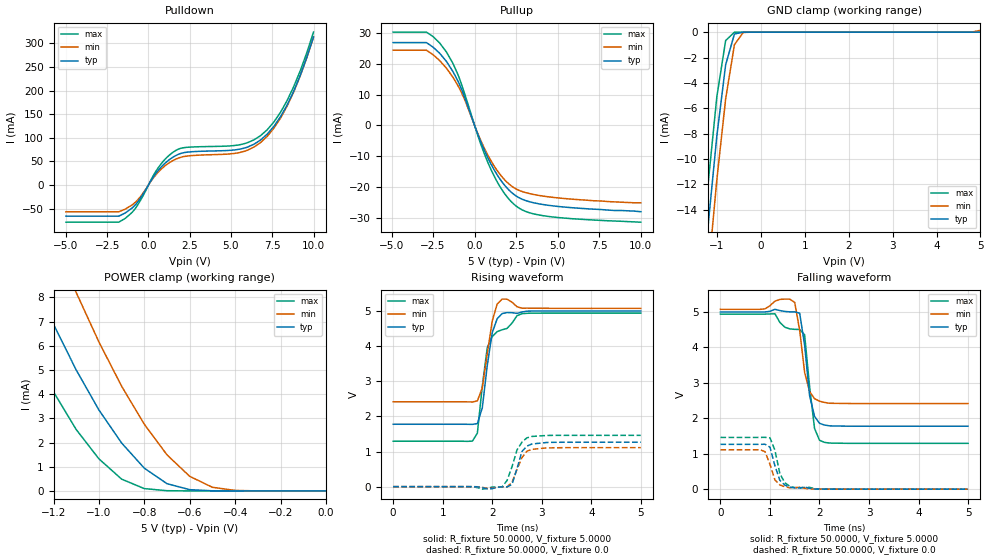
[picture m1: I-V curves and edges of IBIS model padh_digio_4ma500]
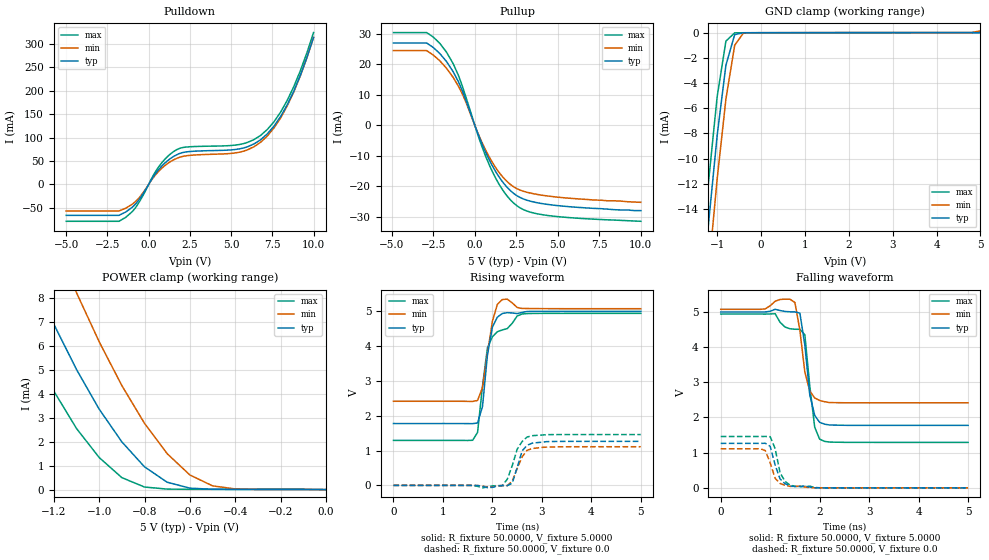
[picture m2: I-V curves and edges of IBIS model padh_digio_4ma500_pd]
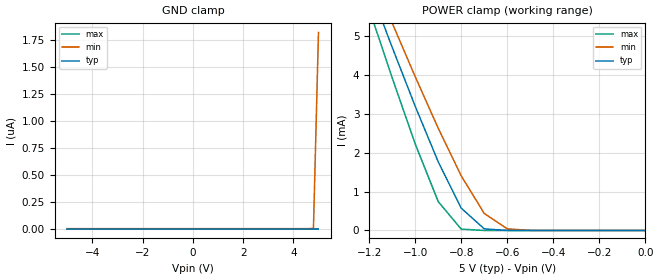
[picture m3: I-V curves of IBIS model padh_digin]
| IBIS file cs4272.ibs created by s2ibis3 verion 1.0
| North Carolina State University, ERL, 2005
[IBIS ver]   3.2
[Comment char]  |_char
[File name]   cs4272.ibs
[File Rev]   1.0B
[Date]   January 26, 2003
[Source]   HSpice Netlist
[Notes]   Rev. 1.0  1/26/2006  28-pin.  Original file.
|   Created by D. DeVries
[Copyright]   (C)opyright 2003 Cirrus Logic, Inc.  All Rights Reserved
[Component]   cs4272
[Manufacturer]  Cirrus Logic, Inc.
|   Component cs4272
[Package]
| variable   typ   min   max
R_pkg   12m   6.8m   16.1m
L_pkg   1.4n   0.713n   2.100n
C_pkg   0.27p   0.180p   0.368p
[Pin]  signal_name   model_name   R_pin   L_pin   C_pin
1   XTO   NC
2   XTI   NC
3   MCLK   padh_digio_mclk_pd
4   LRCK   padh_digio_4ma500
5   SCLK   padh_digio_4ma500
6   SDOUT   padh_digio_4ma500_pd
7   SDIN   padh_digin
8   DGND   GND
9   VD   POWER
10   VL   POWER
11   SCL_CCLK   padh_digin
12   SDA_CDIN   padh_digio_mclk
13   AD0_CSB   padh_digin
14   RSTB   padh_digin
15   VCOM   NC
16   AINA-   NC
17   AINA+   NC
18   AINB+   NC
19   AINB-   NC
20   VA   POWER
21   AGND   GND
22   FILT+   NC
23   AMUTECB   NC
24   AOUTA-   NC
25   AOUTA+   NC
26   AOUTB+   NC
27   AOUTB-   NC
28   BMUTECB   NC
| Models and submodels in the file (5): padh_digio_4ma500 (I/O), padh_digio_4ma500_pd (I/O), padh_digin (Input), padh_digio_mclk (I/O), padh_digio_mclk_pd (I/O)
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|   Model sclk
[Model]  padh_digio_4ma500
Model_type I/O
Polarity   Non-Inverting
Enable   Active-High
Vinl =   0.8000V
Vinh =   2.0000V
C_comp   5.0000pF   5.0000pF   5.0000pF
[Temperature Range]   25.0000   85.0000   -40.0000
[Voltage Range]   5.0000V   4.5000V   5.5000V
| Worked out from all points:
|   slope of the pulldown table from 0 to 0.75 V, typ, clamps not added: 20.1 ohm
|   slope of the pullup table from 0 to 0.75 V, typ, clamps not added: 75.3 ohm
|   GND clamp passes 1 mA (typ) near -0.67 V on its own axis
|   POWER clamp passes 1 mA (typ) near -0.81 V on its own axis
|   rising waveform, R_fixture 50.0000, V_fixture 5.0000: 20-80 % time 183ps typ, 168ps min, 243ps max; typ from 1.78 V to 5 V
|   rising waveform, R_fixture 50.0000, V_fixture 0.0: 20-80 % time 166ps typ, 207ps min, 227ps max; typ from 0 V to 1.26 V
|   falling waveform, R_fixture 50.0000, V_fixture 5.0000: 20-80 % time 170ps typ, 172ps min, 164ps max; typ from 5 V to 1.78 V
|   falling waveform, R_fixture 50.0000, V_fixture 0.0: 20-80 % time 166ps typ, 180ps min, 176ps max; typ from 1.26 V to 0 V
[Pulldown]
|Voltage   I(typ)   I(min)   I(max)
-5V       -65.95mA   -56.72mA   -78.71mA
-1.8V     -65.95mA   -56.72mA   -78.71mA
-900mV    -45.7mA    -39.64mA   -54.33mA
600mV     31.21mA    27.58mA    36.99mA
1.6V      61.37mA    53.94mA    72.04mA
2.4V      69.89mA    61.65mA    80.11mA
5.5V      75.87mA    68.75mA    85.23mA
6.8V      95.63mA    90.28mA    104.9mA
7.6V      124.3mA    120.6mA    133.7mA
8.4V      169.6mA    167.3mA    179.1mA
9.2V      232.7mA    231.7mA    242.5mA
10V       313.7mA    313.6mA    324.1mA
[Pullup]
|Voltage   I(typ)   I(min)   I(max)
-4.9V     26.89mA    24.42mA    30.3mA
-2.9V     26.89mA    24.42mA    30.3mA
-2.1V     23.42mA    21.04mA    26.73mA
-1.7V     20.81mA    18.62mA    23.87mA
-900mV    13.2mA     11.86mA    15.06mA
300mV     -4.326mA   -3.99mA    -4.956mA
900mV     -11.63mA   -10.65mA   -13.28mA
1.7V      -18.69mA   -17.01mA   -21.32mA
2.5V      -22.9mA    -20.63mA   -26.16mA
3.3V      -24.75mA   -22.11mA   -28.33mA
4.6V      -26.03mA   -23.27mA   -29.64mA
10V       -28mA      -25.1mA    -31.4mA
[GND_clamp]
|Voltage   I(typ)   I(min)   I(max)
-5V       -173mA     -172.2mA   -178.6mA
-1.4V     -23.29mA   -27.28mA   -20.11mA
-1.2V     -15.28mA   -19.12mA   -11.98mA
-1V       -8.176mA   -11.63mA   -5.085mA
-800mV    -2.575mA   -5.266mA   -663.9uA
-600mV    -146.2uA   -989.3uA   -4.169uA
-400mV    -717.5nA   -22.85uA   -2.528nA
4.8V      98.24pA    41.38nA    86.34pA
5V        107pA      150uA      94.52pA
[POWER_clamp]
|Voltage   I(typ)   I(min)   I(max)
-5V       117.7mA    125mA      114.4mA
-1.4V     11.23mA    15.35mA    7.972mA
-1.3V     8.971mA    12.82mA    5.918mA
-1.2V     6.884mA    10.43mA    4.093mA
-1.1V     4.997mA    8.198mA    2.536mA
-1V       3.345mA    6.155mA    1.325mA
-900mV    1.981mA    4.328mA    487.2uA
-800mV    939.3uA    2.755mA    95.74uA
-700mV    299uA      1.489mA    9.484uA
-600mV    51.78uA    603.4uA    549nA
-400mV    325.6nA    21.08uA    419.7pA
0V        107pA      1.158nA    115pA
[Ramp]
| variable   typ   min   max
dV/dt_r  0.7590/0.1546n   0.5827/0.1884n   0.9708/0.1428n
dV/dt_f  1.9344/0.1381n   1.5444/0.1722n   2.3550/0.1231n
R_load = 50.0000
[Rising Waveform]
R_fixture= 50.0000
V_fixture= 5.0000
V_fixture_min= 5.5000
V_fixture_max= 4.5000
|time   V(typ)   V(min)   V(max)
0s        1.776V     2.416V     1.293V
1.6ns     1.772V     2.41V      1.296V
1.7ns     1.794V     2.439V     1.522V
1.8ns     2.248V     2.813V     2.867V
1.9ns     3.45V      3.781V     3.961V
2ns       4.383V     4.715V     4.271V
2.1ns     4.78V      5.198V     4.413V
2.2ns     4.926V     5.339V     4.465V
2.6ns     4.971V     5.079V     4.923V
5ns       5V         5.074V     4.94V
[Rising Waveform]
R_fixture= 50.0000
V_fixture= 0.0
|time   V(typ)   V(min)   V(max)
0s        0V         0V         0V
1.8ns     -26.82mV   -20.66mV   -71.47mV
2.2ns     -5.674mV   -5.304mV   -5.196mV
2.3ns     -6.798mV   -6.721mV   176.7mV
2.4ns     63.92mV    122.6mV    567.5mV
2.5ns     512.4mV    491.5mV    1.044V
2.6ns     999.4mV    825.3mV    1.265V
2.7ns     1.154V     1.01V      1.39V
3.1ns     1.257V     1.101V     1.457V
5ns       1.265V     1.11V      1.46V
[Falling Waveform]
R_fixture= 50.0000
V_fixture= 5.0000
V_fixture_min= 5.5000
V_fixture_max= 4.5000
|time   V(typ)   V(min)   V(max)
0s        5V         5.074V     4.94V
1.1ns     5.074V     5.304V     4.949V
1.4ns     5.004V     5.361V     4.522V
1.5ns     5.002V     5.269V     4.509V
1.6ns     4.966V     4.479V     4.506V
1.7ns     4.059V     3.293V     4.353V
1.8ns     2.641V     2.754V     2.894V
1.9ns     2.054V     2.555V     1.714V
2ns       1.859V     2.482V     1.381V
5ns       1.776V     2.416V     1.293V
[Falling Waveform]
R_fixture= 50.0000
V_fixture= 0.0
|time   V(typ)   V(min)   V(max)
0s        1.265V     1.11V      1.46V
800ps     1.264V     1.112V     1.46V
900ps     1.268V     1.058V     1.462V
1ns       1.185V     702.3mV    1.448V
1.1ns     659.7mV    261.3mV    1.099V
1.2ns     248.9mV    119mV      436.1mV
1.3ns     114.2mV    67.55mV    181.8mV
1.5ns     35.29mV    42.46mV    44.87mV
2.1ns     617.8uV    480.5uV    560.9uV
5ns       -7.274uV   0V         3.973uV
|   Model sclk
[Model]  padh_digio_4ma500_pd
Model_type I/O
Polarity   Non-Inverting
Enable   Active-High
Vinl =   0.8000V
Vinh =   2.0000V
C_comp   5.0000pF   5.0000pF   5.0000pF
[Temperature Range]   25.0000   85.0000   -40.0000
[Voltage Range]   5.0000V   4.5000V   5.5000V
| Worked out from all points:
|   slope of the pulldown table from 0 to 0.75 V, typ, clamps not added: 20.1 ohm
|   slope of the pullup table from 0 to 0.75 V, typ, clamps not added: 75.3 ohm
|   GND clamp passes 1 mA (typ) near -0.67 V on its own axis
|   POWER clamp passes 1 mA (typ) near -0.81 V on its own axis
|   rising waveform, R_fixture 50.0000, V_fixture 5.0000: 20-80 % time 165ps typ, 168ps min, 244ps max; typ from 1.78 V to 5 V
|   rising waveform, R_fixture 50.0000, V_fixture 0.0: 20-80 % time 171ps typ, 210ps min, 229ps max; typ from 0 V to 1.26 V
|   falling waveform, R_fixture 50.0000, V_fixture 5.0000: 20-80 % time 171ps typ, 172ps min, 165ps max; typ from 5 V to 1.78 V
|   falling waveform, R_fixture 50.0000, V_fixture 0.0: 20-80 % time 168ps typ, 185ps min, 172ps max; typ from 1.26 V to 0 V
[Pulldown]
|Voltage   I(typ)   I(min)   I(max)
-5V       -66.04mA   -56.71mA   -78.7mA
-1.8V     -66.04mA   -56.71mA   -78.7mA
-900mV    -45.69mA   -39.64mA   -54.33mA
600mV     31.21mA    27.58mA    36.99mA
1.6V      61.37mA    53.95mA    72.04mA
2.4V      69.89mA    61.65mA    80.11mA
5.5V      75.88mA    68.76mA    85.23mA
6.8V      95.62mA    90.28mA    104.9mA
7.6V      124.3mA    120.6mA    133.7mA
8.4V      169.6mA    167.3mA    179.1mA
9.2V      232.7mA    231.7mA    242.6mA
10V       313.7mA    313.6mA    324.1mA
[Pullup]
|Voltage   I(typ)   I(min)   I(max)
-4.9V     26.89mA    24.41mA    30.31mA
-2.9V     26.89mA    24.41mA    30.31mA
-2.1V     23.42mA    21.04mA    26.73mA
-1.7V     20.81mA    18.61mA    23.87mA
-900mV    13.2mA     11.87mA    15.06mA
300mV     -4.325mA   -3.99mA    -4.956mA
900mV     -11.63mA   -10.66mA   -13.28mA
1.7V      -18.69mA   -17.01mA   -21.31mA
2.5V      -22.9mA    -20.63mA   -26.16mA
3.2V      -24.6mA    -21.98mA   -28.16mA
4.4V      -25.89mA   -23.14mA   -29.51mA
10V       -27.9mA    -25.2mA    -31.4mA
[GND_clamp]
|Voltage   I(typ)   I(min)   I(max)
-5V       -173.1mA   -172.2mA   -178.6mA
-1.4V     -23.3mA    -27.29mA   -20.11mA
-1.2V     -15.29mA   -19.13mA   -11.99mA
-1V       -8.181mA   -11.63mA   -5.091mA
-800mV    -2.579mA   -5.27mA    -668.7uA
-600mV    -149.1uA   -991.8uA   -7.709uA
-400mV    -2.632uA   -24.53uA   -2.341uA
4.8V      8.423uA    6.634uA    11.35uA
5V        8.425uA    156.6uA    11.35uA
[POWER_clamp]
|Voltage   I(typ)   I(min)   I(max)
-5V       117.7mA    125mA      114.4mA
-1.4V     11.24mA    15.35mA    7.983mA
-1.3V     8.979mA    12.82mA    5.93mA
-1.2V     6.892mA    10.43mA    4.104mA
-1.1V     5.006mA    8.205mA    2.547mA
-1V       3.353mA    6.161mA    1.337mA
-900mV    1.99mA     4.334mA    498.5uA
-800mV    947.7uA    2.762mA    107.1uA
-700mV    307.4uA    1.496mA    20.85uA
-600mV    60.22uA    609.9uA    11.92uA
-400mV    8.755uA    27.67uA    11.37uA
0V        0A         0A         0A
[Ramp]
| variable   typ   min   max
dV/dt_r  0.7584/0.1574n   0.5825/0.1726n   0.9702/0.1477n
dV/dt_f  1.9338/0.1385n   1.5438/0.1725n   2.3544/0.1238n
R_load = 50.0000
[Rising Waveform]
R_fixture= 50.0000
V_fixture= 5.0000
V_fixture_min= 5.5000
V_fixture_max= 4.5000
|time   V(typ)   V(min)   V(max)
0s        1.776V     2.416V     1.292V
1.6ns     1.772V     2.41V      1.296V
1.7ns     1.794V     2.439V     1.52V
1.8ns     2.264V     2.812V     2.852V
1.9ns     3.749V     3.78V      3.954V
2ns       4.546V     4.714V     4.268V
2.1ns     4.83V      5.197V     4.412V
2.2ns     4.936V     5.337V     4.464V
2.6ns     4.968V     5.08V      4.923V
5ns       4.999V     5.074V     4.94V
[Rising Waveform]
R_fixture= 50.0000
V_fixture= 0.0
|time   V(typ)   V(min)   V(max)
0s        0V         0V         0V
1.8ns     -26.6mV    -20.45mV   -70.99mV
2.2ns     -5.958mV   -5.588mV   -5.25mV
2.3ns     -6.889mV   -6.797mV   174.2mV
2.4ns     62.49mV    120mV      560.7mV
2.5ns     504.2mV    483mV      1.035V
2.6ns     987.8mV    815.9mV    1.258V
2.7ns     1.149V     1.006V     1.387V
3.1ns     1.256V     1.099V     1.457V
5ns       1.264V     1.11V      1.46V
[Falling Waveform]
R_fixture= 50.0000
V_fixture= 5.0000
V_fixture_min= 5.5000
V_fixture_max= 4.5000
|time   V(typ)   V(min)   V(max)
0s        4.999V     5.074V     4.94V
1.1ns     5.074V     5.304V     4.949V
1.4ns     5.004V     5.361V     4.522V
1.5ns     5.001V     5.269V     4.508V
1.6ns     4.966V     4.479V     4.506V
1.7ns     4.059V     3.293V     4.352V
1.8ns     2.645V     2.754V     2.899V
1.9ns     2.059V     2.555V     1.722V
2ns       1.861V     2.482V     1.383V
5ns       1.776V     2.416V     1.292V
[Falling Waveform]
R_fixture= 50.0000
V_fixture= 0.0
|time   V(typ)   V(min)   V(max)
0s        1.264V     1.11V      1.46V
800ps     1.264V     1.112V     1.46V
900ps     1.268V     1.06V      1.462V
1ns       1.18V      709.5mV    1.454V
1.1ns     648.2mV    271.8mV    1.111V
1.2ns     251.8mV    125mV      430.1mV
1.3ns     117.3mV    70.64mV    182.3mV
1.5ns     35.44mV    42.99mV    43.95mV
1.9ns     2.19mV     1.683mV    11.88mV
5ns       -5.401uV   -1.059uV   -26.02uV
|   Model padh_digin
[Model]  padh_digin
Model_type Input
Vinl =   0.8000V
Vinh =   2.0000V
C_comp   5.0000pF   5.0000pF   5.0000pF
[Temperature Range]   25.0000   85.0000   -40.0000
[Voltage Range]   5.0000V   4.5000V   5.5000V
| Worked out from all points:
|   POWER clamp passes 1 mA (typ) near -0.84 V on its own axis
[GND_clamp]
|Voltage   I(typ)   I(min)   I(max)
-5V       -30pA      -28.67pA   -31.5pA
4.6V      -1.2pA     178.1fA    -2.7pA
4.8V      -600.1fA   2.835nA    -2.1pA
5V        0A         1.821uA    -1.5pA
[POWER_clamp]
|Voltage   I(typ)   I(min)   I(max)
-5V       69.3mA     63.46mA    77.41mA
-1.2V     6.274mA    6.747mA    5.694mA
-1.1V     4.711mA    5.337mA    3.925mA
-1V       3.195mA    3.956mA    2.226mA
-900mV    1.764mA    2.629mA    741.3uA
-800mV    572.3uA    1.403mA    34.11uA
-700mV    41.8uA     437uA      266.3nA
-600mV    967.8nA    41.61uA    1.853nA
-500mV    19.92nA    1.821uA    14.35pA
0V        0A         0A         0A
